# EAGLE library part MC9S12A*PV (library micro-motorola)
MC9S12A256 microcontroller unit (MCU) 16-bit HCS12 Core; Upward compatible with M68HC11 instruction set Source: 9S12A128DGV1.pdf; 9S12A256DGV1.pdf
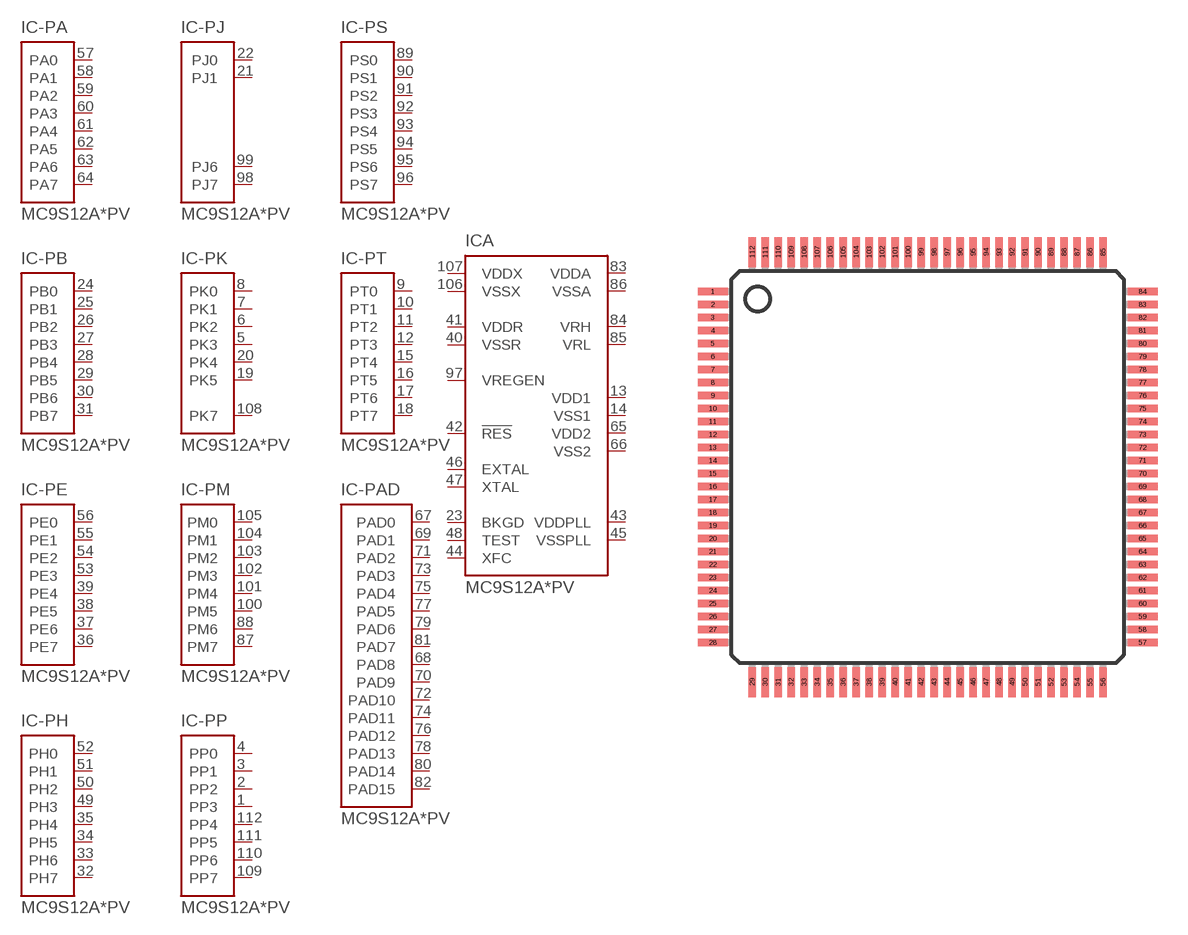
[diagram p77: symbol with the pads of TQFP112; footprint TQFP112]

Designator prefix IC; gates -PA=MC9S12-PA -PB=MC9S12-PB -PE=MC9S12-PE -PP=MC9S12-PP -PM=MC9S12-PM -PS=MC9S12-PS -PT=MC9S12-PT -PH=MC9S12-PH -PAD=MC9S12-PADAN15 -PK=MC9S12-PK -PJ=MC9S12-PJ A=MC9S12A256

## MC9S12A128BCPV (MF: MOTOROLA; MPN: MC9S12A128CPV; OC_FARNELL: unknown; OC_NEWARK: 86H4601), MC9S12A256CPV (MPN: MC9S12A256CPVE; OC_FARNELL: 1165785; OC_NEWARK: 70K3218)  [TQFP112]
1  -PP:PP3
2  -PP:PP2
3  -PP:PP1
4  -PP:PP0
5  -PK:PK3
6  -PK:PK2
7  -PK:PK1
8  -PK:PK0
9  -PT:PT0
10  -PT:PT1
11  -PT:PT2
12  -PT:PT3
13  A:VDD1  out
14  A:VSS1  out
15  -PT:PT4
16  -PT:PT5
17  -PT:PT6
18  -PT:PT7
19  -PK:PK5
20  -PK:PK4
21  -PJ:PJ1
22  -PJ:PJ0
23  A:BKGD  oc
24  -PB:PB0
25  -PB:PB1
26  -PB:PB2
27  -PB:PB3
28  -PB:PB4
29  -PB:PB5
30  -PB:PB6
31  -PB:PB7
32  -PH:PH7
33  -PH:PH6
34  -PH:PH5
35  -PH:PH4
36  -PE:PE7
37  -PE:PE6
38  -PE:PE5
39  -PE:PE4
40  A:VSSR  pwr
41  A:VDDR  pwr
42  A:!RES
43  A:VDDPLL  out
44  A:XFC
45  A:VSSPLL  out
46  A:EXTAL  in
47  A:XTAL  out
48  A:TEST  in
49  -PH:PH3
50  -PH:PH2
51  -PH:PH1
52  -PH:PH0
53  -PE:PE3
54  -PE:PE2
55  -PE:PE1  in
56  -PE:PE0  in
57  -PA:PA0
58  -PA:PA1
59  -PA:PA2
60  -PA:PA3
61  -PA:PA4
62  -PA:PA5
63  -PA:PA6
64  -PA:PA7
65  A:VDD2  out
66  A:VSS2  out
67  -PAD:PAD0  in
68  -PAD:PAD8  in
69  -PAD:PAD1  in
70  -PAD:PAD9  in
71  -PAD:PAD2  in
72  -PAD:PAD10  in
73  -PAD:PAD3  in
74  -PAD:PAD11  in
75  -PAD:PAD4  in
76  -PAD:PAD12  in
77  -PAD:PAD5  in
78  -PAD:PAD13  in
79  -PAD:PAD6  in
80  -PAD:PAD14  in
81  -PAD:PAD7  in
82  -PAD:PAD15  in
83  A:VDDA  pwr
84  A:VRH  in
85  A:VRL  in
86  A:VSSA  pwr
87  -PM:PM7
88  -PM:PM6
89  -PS:PS0
90  -PS:PS1
91  -PS:PS2
92  -PS:PS3
93  -PS:PS4
94  -PS:PS5
95  -PS:PS6
96  -PS:PS7
97  A:VREGEN  in
98  -PJ:PJ7
99  -PJ:PJ6
100  -PM:PM5
101  -PM:PM4
102  -PM:PM3
103  -PM:PM2
104  -PM:PM1
105  -PM:PM0
106  A:VSSX  pwr
107  A:VDDX  pwr
108  -PK:PK7
109  -PP:PP7
110  -PP:PP6
111  -PP:PP5
112  -PP:PP4

## Footprint TQFP112 (pad centres in mm)
Thin Quad Flat Pack 112-Pin LQFP (Case no. 987) 9S12A256DGV1.pdf
smd 1.5 x 0.37: 1 -10.75,8.775; 2 -10.75,8.125; 3 -10.75,7.475; 4 -10.75,6.825; 5 -10.75,6.175; 6 -10.75,5.525; 7 -10.75,4.875; 8 -10.75,4.225; 9 -10.75,3.575; 10 -10.75,2.925; 11 -10.75,2.275; 12 -10.75,1.625; 13 -10.75,0.975; 14 -10.75,0.325; 15 -10.75,-0.325; 16 -10.75,-0.975; 17 -10.75,-1.625; 18 -10.75,-2.275; 19 -10.75,-2.925; 20 -10.75,-3.575; 21 -10.75,-4.225; 22 -10.75,-4.875; 23 -10.75,-5.525; 24 -10.75,-6.175; 25 -10.75,-6.825; 26 -10.75,-7.475; 27 -10.75,-8.125; 28 -10.75,-8.775; 57 10.75,-8.775; 58 10.75,-8.125; 59 10.75,-7.475; 60 10.75,-6.825; 61 10.75,-6.175; 62 10.75,-5.525; 63 10.75,-4.875; 64 10.75,-4.225; 65 10.75,-3.575; 66 10.75,-2.925; 67 10.75,-2.275; 68 10.75,-1.625; 69 10.75,-0.975; 70 10.75,-0.325; 71 10.75,0.325; 72 10.75,0.975; 73 10.75,1.625; 74 10.75,2.275; 75 10.75,2.925; 76 10.75,3.575; 77 10.75,4.225; 78 10.75,4.875; 79 10.75,5.525; 80 10.75,6.175; 81 10.75,6.825; 82 10.75,7.475; 83 10.75,8.125; 84 10.75,8.775
smd 0.37 x 1.5: 29 -8.775,-10.75; 30 -8.125,-10.75; 31 -7.475,-10.75; 32 -6.825,-10.75; 33 -6.175,-10.75; 34 -5.525,-10.75; 35 -4.875,-10.75; 36 -4.225,-10.75; 37 -3.575,-10.75; 38 -2.925,-10.75; 39 -2.275,-10.75; 40 -1.625,-10.75; 41 -0.975,-10.75; 42 -0.325,-10.75; 43 0.325,-10.75; 44 0.975,-10.75; 45 1.625,-10.75; 46 2.275,-10.75; 47 2.925,-10.75; 48 3.575,-10.75; 49 4.225,-10.75; 50 4.875,-10.75; 51 5.525,-10.75; 52 6.175,-10.75; 53 6.825,-10.75; 54 7.475,-10.75; 55 8.125,-10.75; 56 8.775,-10.75; 85 8.775,10.75; 86 8.125,10.75; 87 7.475,10.75; 88 6.825,10.75; 89 6.175,10.75; 90 5.525,10.75; 91 4.875,10.75; 92 4.225,10.75; 93 3.575,10.75; 94 2.925,10.75; 95 2.275,10.75; 96 1.625,10.75; 97 0.975,10.75; 98 0.325,10.75; 99 -0.325,10.75; 100 -0.975,10.75; 101 -1.625,10.75; 102 -2.275,10.75; 103 -2.925,10.75; 104 -3.575,10.75; 105 -4.225,10.75; 106 -4.875,10.75; 107 -5.525,10.75; 108 -6.175,10.75; 109 -6.825,10.75; 110 -7.475,10.75; 111 -8.125,10.75; 112 -8.775,10.75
